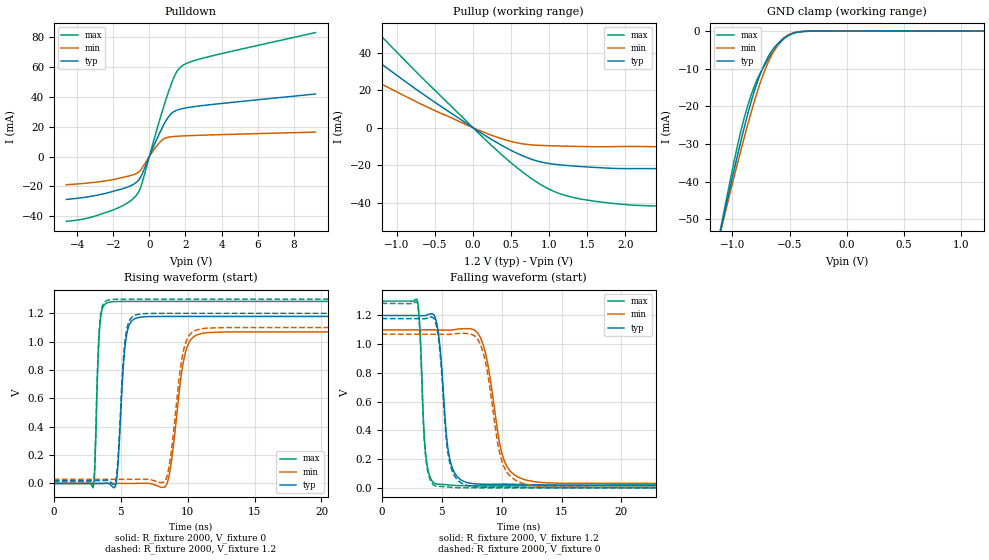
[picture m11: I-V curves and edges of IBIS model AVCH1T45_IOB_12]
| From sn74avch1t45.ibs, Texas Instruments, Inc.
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[Model]   AVCH1T45_IOB_12
Model_type  I/O
Vinl=0.385
Vinh=0.845
Enable   Active-High
Vref =   0
Rref =   2000
Cref =   15p
Vmeas =   0.6
| variable   typ   min   max
C_comp   5.41pF   4.77pF   5.94pF
| C_pullup   5.90pF   3.97pF   7.94pF
| C_pulldown   5.45pF   4.81pF   7.14pF
| C_tri-state   5.41pF   4.77pF   5.94pF
[Temperature Range]   40   100   -40
| Ambient temperature   25   85   -40
[Voltage range]   1.2   1.1   1.3
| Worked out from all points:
|   slope of the pulldown table from 0 to 0.18 V, typ, clamps not added: 34.6 ohm
|   slope of the pullup table from 0 to 0.18 V, typ, clamps not added: 38.6 ohm
|   GND clamp passes 1 mA (typ) near -0.50 V on its own axis
|   rising waveform, R_fixture 2000, V_fixture 0: 20-80 % time 434ps typ, 807ps min, 264ps max; typ from 0 V to 1.18 V
|   falling waveform, R_fixture 2000, V_fixture 1.2: 20-80 % time 678ps typ, 1.23ns min, 404ps max; typ from 1.2 V to 0.02 V
|   rising waveform, R_fixture 2000, V_fixture 1.2: 20-80 % time 427ps typ, 782ps min, 261ps max; typ from 0.02 V to 1.2 V
|   falling waveform, R_fixture 2000, V_fixture 0: 20-80 % time 676ps typ, 1.22ns min, 402ps max; typ from 1.18 V to 0 V
[GND Clamp]
| AVCH1T45_IOB_12
|   Voltage   I(typ)   I(min)   I(max)
-4.6V     -599.5mA   -548.1mA   -664.5mA
-1.095V   -51.65mA   -52.16mA   -51.03mA
-1.07V    -48.2mA    -49.03mA   -47.15mA
-940mV    -30.92mA   -33.24mA   -28.27mA
-840mV    -19.11mA   -21.95mA   -17.27mA
-775mV    -12.93mA   -15.39mA   -12.23mA
-695mV    -7.282mA   -8.82mA    -7.866mA
-615mV    -3.733mA   -4.168mA   -4.305mA
-545mV    -1.871mA   -1.692mA   -1.969mA
-465mV    -604.4uA   -486.8uA   -527.9uA
-355mV    -86uA      -70.97uA   -92.21uA
1.2V      714.8pA    8.498uA    -20.59uA
[Pulldown]
| AVCH1T45_IOB_12
|   Voltage   I(typ)   I(min)   I(max)
-4.6V     -28.79mA   -18.92mA   -43.46mA
-3.415V   -27.06mA   -17.81mA   -41.32mA
-2.035V   -23.45mA   -15.53mA   -35.96mA
-1.17V    -20.3mA    -13.14mA   -30.86mA
-680mV    -16.87mA   -11.13mA   -25.38mA
-435mV    -12.68mA   -8.327mA   -19.06mA
440mV     12.38mA    7.543mA    19.04mA
955mV     24.67mA    12.69mA    39.57mA
1.42V     30.53mA    13.49mA    54.64mA
1.79V     32.04mA    13.78mA    60.61mA
3.17V     34.51mA    14.41mA    66.63mA
9.2V      41.96mA    16.4mA     83.17mA
[Pullup]
| AVCH1T45_IOB_12
|   Voltage   I(typ)   I(min)   I(max)
-4.6V     40.24mA    7.956mA    186.3mA
-4.08V    45.4mA     8.808mA    167.8mA
-3.73V    53.62mA    9.647mA    154.2mA
-2.685V   79.31mA    16.98mA    111.4mA
-2.57V    75.87mA    21.96mA    106.5mA
-2.565V   75.72mA    49.42mA    106.3mA
-1.845V   53.66mA    37.03mA    75.82mA
-1.36V    38.76mA    26.71mA    55.3mA
575mV     -13.51mA   -7.977mA   -21.19mA
1.01V     -19.08mA   -9.527mA   -32.92mA
1.455V    -20.71mA   -9.971mA   -38.21mA
9.2V      -28.28mA   -12.48mA   -52.65mA
[Ramp]
| AVCH1T45_IOB_12
| variable   typ   min   max
dV/dt_r   0.72/4.48E-10   0.66/8.26E-10   0.79/2.79E-10
dV/dt_f   0.72/6.85E-10   0.65/1.24E-09   0.78/4.10E-10
R_load = 2000
[Rising Waveform]
| AVCH1T45_IOB_12
R_fixture =   2000
C_fixture =   0
L_fixture =   0
V_fixture =   0
V_fixture_min = 0
V_fixture_max = 0
|   Time   V(typ)   V(min)   V(max)
0s        18.14nV    102.1nV    431.7pV
2.935ns   8.857uV    927.6nV    -26.34mV
3.435ns   -98.87uV   -3.229uV   1.111V
4.005ns   1.977mV    6.863uV    1.274V
4.655ns   471.9uV    4.853uV    1.283V
5.34ns    982.9mV    -48.64uV   1.284V
6.12ns    1.165V     121.9uV    1.284V
8.455ns   1.178V     -1.266mV   1.284V
10.72ns   1.178V     1.049V     1.284V
34.99ns   1.178V     1.069V     1.284V
[Falling Waveform]
| AVCH1T45_IOB_12
R_fixture =   2000
C_fixture =   0
L_fixture =   0
V_fixture =   1.2
V_fixture_min = 1.1
V_fixture_max = 1.3
|   Time   V(typ)   V(min)   V(max)
0s        1.2V       1.1V       1.3V
2.955ns   1.2V       1.1V       1.308V
3.655ns   1.2V       1.1V       242.2mV
4.45ns    1.188V     1.1V       29.87mV
5.6ns     232.7mV    1.098V     20.25mV
6.815ns   45.98mV    1.108V     15.12mV
8.365ns   25.53mV    1.019V     14.48mV
10.04ns   25.79mV    236.1mV    14.45mV
11.49ns   23.97mV    70.3mV     14.45mV
34.99ns   20.07mV    28.68mV    14.44mV
[Rising Waveform]
| AVCH1T45_IOB_12
R_fixture =   2000
C_fixture =   0
L_fixture =   0
V_fixture =   1.2
V_fixture_min = 1.1
V_fixture_max = 1.3
|   Time   V(typ)   V(min)   V(max)
0s        20.07mV    28.66mV    14.44mV
2.93ns    20.08mV    28.66mV    -12.19mV
3.425ns   19.98mV    28.66mV    1.123V
3.975ns   22.08mV    28.67mV    1.291V
4.655ns   30.32mV    28.67mV    1.299V
5.32ns    1.008V     28.62mV    1.3V
6.095ns   1.188V     28.75mV    1.3V
8.385ns   1.2V       32.5mV     1.3V
10.61ns   1.2V       1.081V     1.3V
34.99ns   1.2V       1.1V       1.3V
[Falling Waveform]
| AVCH1T45_IOB_12
R_fixture =   2000
C_fixture =   0
L_fixture =   0
V_fixture =   0
V_fixture_min = 0
V_fixture_max = 0
|   Time   V(typ)   V(min)   V(max)
0s        1.178V     1.069V     1.284V
2.955ns   1.178V     1.069V     1.291V
3.645ns   1.178V     1.069V     231.9mV
4.405ns   1.171V     1.069V     16.42mV
5.585ns   211.7mV    1.068V     5.258mV
6.81ns    26.16mV    1.076V     560.7uV
8.3ns     5.663mV    983.4mV    38.82uV
9.94ns    5.758mV    209.4mV    8.382uV
11.43ns   3.667mV    41.6mV     2.687uV
34.99ns   96.52nV    12.52uV    23.25nV
